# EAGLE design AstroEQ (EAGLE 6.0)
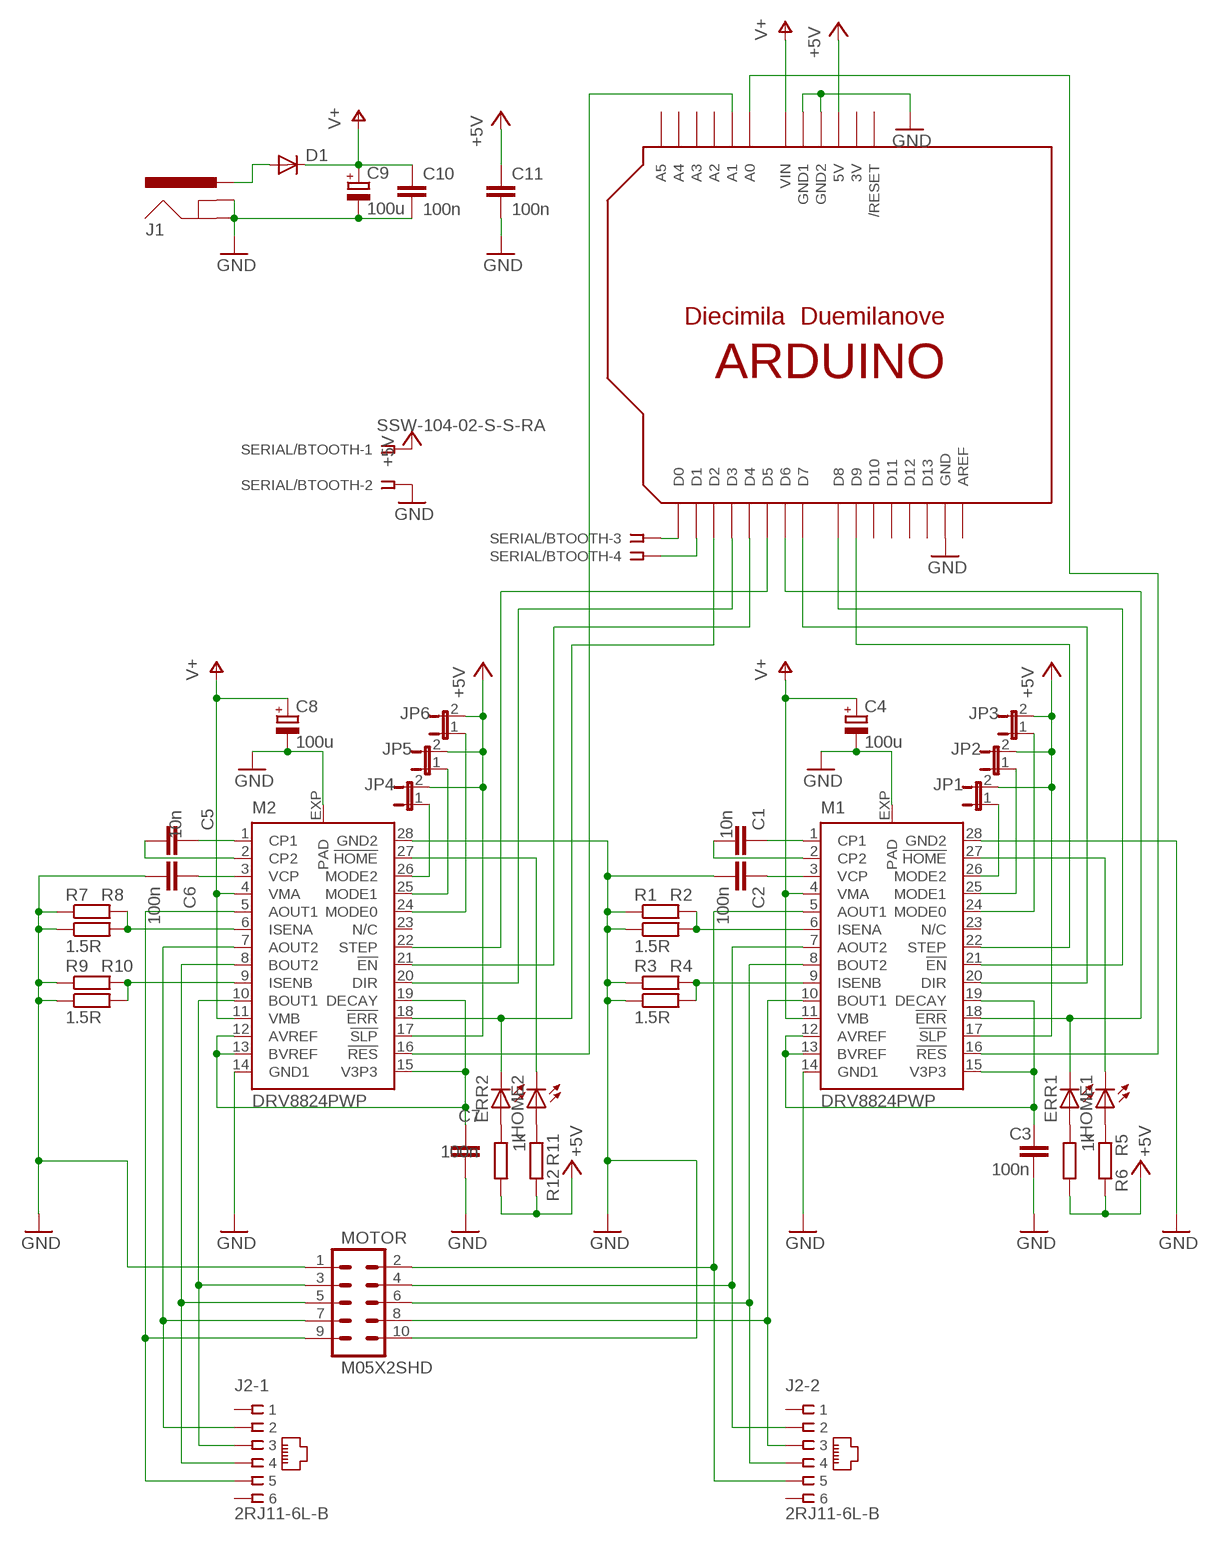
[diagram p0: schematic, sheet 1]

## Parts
C1  10n  C-EUC0603K  [C0603K]
C2  100n  C-EUC0603K  [C0603K]
C3  100n  C-EUC0603K  [C0603K]
C4  100u  CPOL-EUC/6032-28R  [C/6032-28R]
C5  10n  C-EUC0603K  [C0603K]
C6  100n  C-EUC0603K  [C0603K]
C7  100n  C-EUC0603K  [C0603K]
C8  100u  CPOL-EUC/6032-28R  [C/6032-28R]
C9  100u  CPOL-EUC/6032-28R  [C/6032-28R]
C10  100n  C-EUC0603K  [C0603K]
C11  100n  C-EUC0603K  [C0603K]
D1  DIODESMA-ALT  [SMA-DIODE_ALT]
ERR1  LEDCHIP-LED0603  [CHIP-LED0603]
ERR2  LEDCHIP-LED0603  [CHIP-LED0603]
HOME1  LEDCHIP-LED0603  [CHIP-LED0603]
HOME2  LEDCHIP-LED0603  [CHIP-LED0603]
J1  POWER_JACKPTH  [POWER_JACK_PTH]
J2  2RJ11-6L-B  [2RJ11]
JP1  JUMPER-2SMD-NO  [SJ_2S-NO]
JP2  JUMPER-2SMD-NO  [SJ_2S-NO]
JP3  JUMPER-2SMD-NO  [SJ_2S-NO]
JP4  JUMPER-2SMD-NO  [SJ_2S-NO]
JP5  JUMPER-2SMD-NO  [SJ_2S-NO]
JP6  JUMPER-2SMD-NO  [SJ_2S-NO]
M1  DRV8824PWP  [HTSSOP28PWP]
M2  DRV8824PWP  [HTSSOP28PWP]
MOTOR  M05X2SHD  [2X5-SHROUDED]
R1  1.5R  R-EU_R2512  [R2512]
R2  1.5R  R-EU_R2512  [R2512]
R3  1.5R  R-EU_R2512  [R2512]
R4  1.5R  R-EU_R2512  [R2512]
R5  1k  R-EU_R0603  [R0603]
R6  1k  R-EU_R0603  [R0603]
R7  1.5R  R-EU_R2512  [R2512]
R8  1.5R  R-EU_R2512  [R2512]
R9  1.5R  R-EU_R2512  [R2512]
R10  1.5R  R-EU_R2512  [R2512]
R11  1k  R-EU_R0603  [R0603]
R12  1k  R-EU_R0603  [R0603]
SERIAL/BTOOTH  SSW-104-02-S-S-RA  [SSW-104-02-S-S-RA]
U$1  ARDUINOUNO  [ARDUINO]

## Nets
3.3V-1: C3.1 M1.12(AVREF) M1.13(BVREF) M1.15(V3P3) M1.19(DECAY)
3.3V-2: C7.1 M2.12(AVREF) M2.13(BVREF) M2.15(V3P3) M2.19(DECAY)
!EN-1: M1.21(!EN) U$1.D8
!EN-2: M2.21(!EN) U$1.D4
!ERR-1: M1.16(!RES) U$1.A0
!ERR-2: ERR2.C M2.18(!ERR) U$1.D2
!HOME-1: HOME1.C M1.27(!HOME)
!HOME-2: HOME2.C M2.27(!HOME)
!RST-1: ERR1.C M1.18(!ERR) U$1.D6
!RST-2: M2.16(!RES) U$1.A1
+5V: C11.1 JP1.2 JP2.2 JP3.2 JP4.2 JP5.2 JP6.2 M1.17(!SLP) M2.17(!SLP) R5.2 R6.2 R11.2 R12.2 SERIAL/BTOOTH.1 U$1.5V
A1-1: J2.2-5 M1.5(AOUT1) MOTOR.2
A1-2: J2.1-5 M2.5(AOUT1) MOTOR.9
A2-1: J2.2-2 M1.7(AOUT2) MOTOR.4
A2-2: J2.1-2 M2.7(AOUT2) MOTOR.7
B1-1: J2.2-3 M1.10(BOUT1) MOTOR.8
B1-2: J2.1-3 M2.10(BOUT1) MOTOR.3
B2-1: J2.2-4 M1.8(BOUT2) MOTOR.6
B2-2: J2.1-4 M2.8(BOUT2) MOTOR.5
CP1-1: C1.1 M1.1(CP1)
CP1-2: C5.1 M2.1(CP1)
CP2-1: C1.2 M1.2(CP2)
CP2-2: C5.2 M2.2(CP2)
DIR-1: M1.20(DIR) U$1.D7
DIR-2: M2.20(DIR) U$1.D3
GND: C2.2 C3.2 C4.- C6.2 C7.2 C8.- C9.- C10.2 C11.2 J1.GND J1.GNDBREAK M1.14(GND1) M1.28(GND2) M1.EXP(PAD) M2.14(GND1) M2.28(GND2) M2.EXP(PAD) MOTOR.1 MOTOR.10 R1.1 R2.1 R3.1 R4.1 R7.1 R8.1 R9.1 R10.1 SERIAL/BTOOTH.2 U$1.GND U$1.GND1 U$1.GND2
ISENA-1: M1.6(ISENA) R1.2 R2.2
ISENA-2: M2.6(ISENA) R7.2 R8.2
ISENB-1: M1.9(ISENB) R3.2 R4.2
ISENB-2: M2.9(ISENB) R9.2 R10.2
LED1: ERR1.A R6.1
LED2: HOME1.A R5.1
LED3: ERR2.A R12.1
LED4: HOME2.A R11.1
M0-1: JP3.1 M1.24(MODE0)
M0-2: JP6.1 M2.24(MODE0)
M1-1: JP2.1 M1.25(MODE1)
M1-2: JP5.1 M2.25(MODE1)
M2-1: JP1.1 M1.26(MODE2)
M2-2: JP4.1 M2.26(MODE2)
N$7: D1.A J1.PWR
RX: SERIAL/BTOOTH.3 U$1.D0
STEP-1: M1.22(STEP) U$1.D9
STEP-2: M2.22(STEP) U$1.D5
TX: SERIAL/BTOOTH.4 U$1.D1
V+: C4.+ C8.+ C9.+ C10.1 D1.C M1.4(VMA) M1.11(VMB) M2.4(VMA) M2.11(VMB) U$1.VIN
VCP-1: C2.1 M1.3(VCP)
VCP-2: C6.1 M2.3(VCP)
Unconnected: J2.1-1 J2.1-6 J2.2-1 J2.2-6 M1.23(N/C) M2.23(N/C) U$1.A2 U$1.A3 U$1.A4 U$1.A5 U$1.AREF U$1.D10 U$1.D11 U$1.D12 U$1.D13 U$1.RESET(/RESET)

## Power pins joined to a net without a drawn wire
3V: U$1.3V

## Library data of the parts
C1-C3 C5-C7 C10 C11 = resistor:C-EU: CAPACITOR, European symbol
C4 C8 C9 = resistor:CPOL-EU: POLARIZED CAPACITOR, European symbol
D1 = SparkFun:DIODE: Diode
ERR1 ERR2 HOME1 HOME2 = led:LED: LED
J1 = SparkFun:POWER_JACK: Power Jack This is the standard 5.5mm barrel jack for power. The PTH is the most common, proven, reliable, footprint. All others are experimental. The Slot footprint only works if the mill layer is transmitted to the PCB fab house so be warned. Spark Fun Electronics SKU : PRT-00119. Mating wall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
J2 = con-tycoelectronics:2RJ11-6L-B: CORCOM Modular RJ Jacks L - Ganged Series Source: www.tycoelectronics.com .. ENG_DS_1654001_1099_RJ_L_0507.pdf; MF: TYCO ELECTRONICS; MPN: 2RJ11-6L-B; OC_FARNELL: unknown; OC_NEWARK: 48F3954
JP1-JP6 = SparkFun:JUMPER-2: Jumper
M1 M2 = texas:DRV8824
MOTOR = SparkFun:M05X2: Header 5x2 Standard 10-pin dual row 0.1" header. Commonly used with AVR-ISP. Use with Spark Fun Electronics SKU: PRT-00778
R1-R12 = resistor:R-EU_: RESISTOR, European symbol
SERIAL/BTOOTH = con-samtec:SSW-104-02-S-S: THROUGH-HOLE .025" SQ POST SOCKET Source: Samtec SSW.pdf; MPN: SSW-104-02-S-S-RA; OC_FARNELL: unknown; OC_NEWARK: 11P9385
U$1 = adafruit:ARDUINO: Arduino Diecimila/Duemilanove Make a shield with ease, this package has all the named pins as well as the two mounting drill holes and an outline of the USB and DC power connector. The outline is on the DIMENSION layer, so if your board house uses it they will cut the outline to match.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

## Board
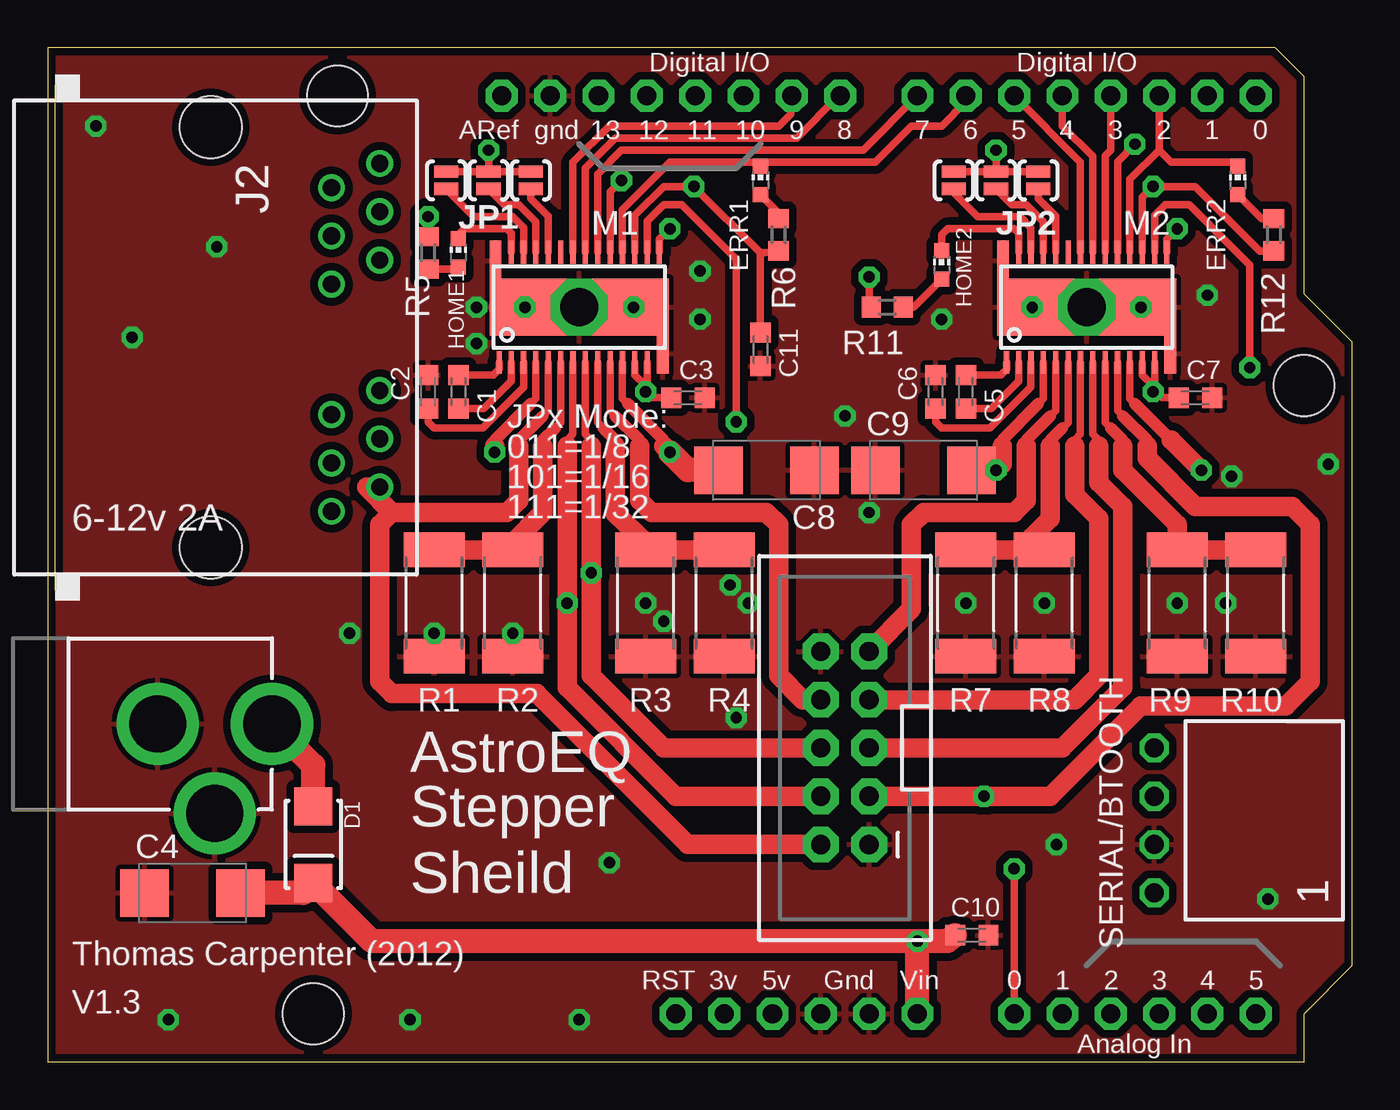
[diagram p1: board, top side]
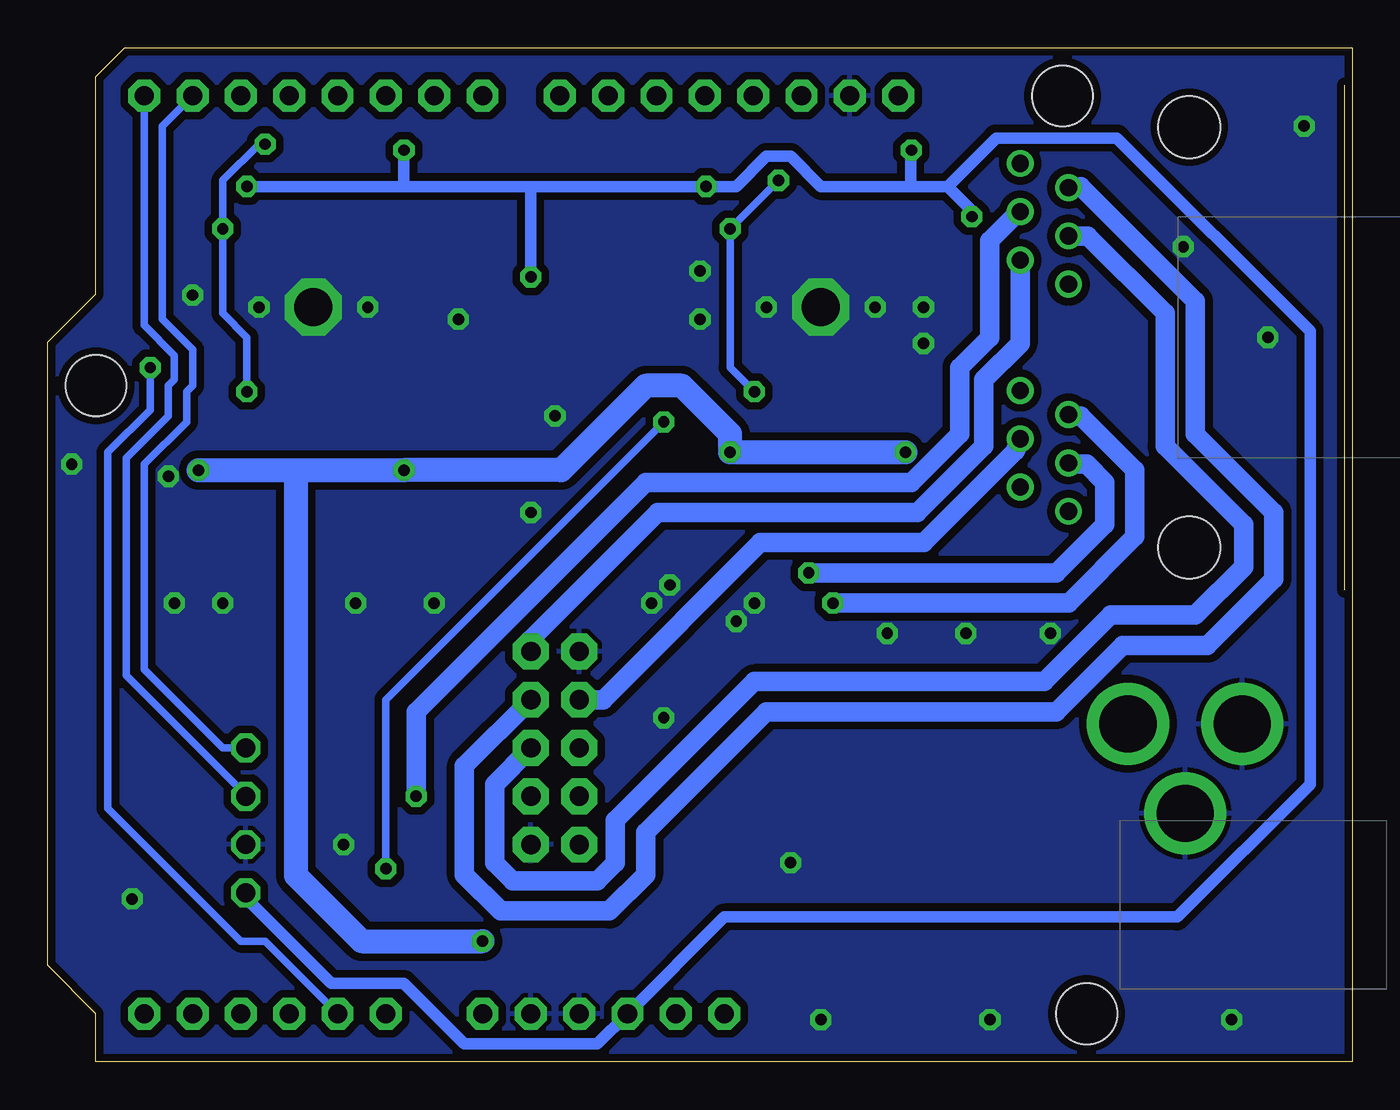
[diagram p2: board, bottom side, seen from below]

Size 68.58 x 53.34 mm. Coordinates in mm from the lower left corner, seen from the top.
Copper layers (1*16): Top 0.035mm / dielectric 1.5mm / Bottom 0.035mm
Design rules: minimum track width 0.2mm, minimum drill 0.4mm, track to track 0.2mm, track to pad 0.2mm, pad to pad 0.2mm, via to via 0.2mm, smd to smd 0mil, copper to edge 10mil, drill to drill 0.2mm, minimum pad ring 10mil, minimum via ring 10mil, stop-mask expansion 0.125mm, vias tented up to drill 0mil, thermal gap 10mil

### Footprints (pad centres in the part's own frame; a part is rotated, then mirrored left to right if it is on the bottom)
C0603K = smd 1.05 x 1.08: 1 -0.875,0; 2 0.875,0
C/6032-28R = smd 2.55 x 2.5: + 2.525,0; - -2.525,0
SMA-DIODE_ALT = smd 2 x 2: A -2,0; C 2,0
CHIP-LED0603 = smd 0.8 x 0.8: A 0,-0.75; C 0,0.75
POWER_JACK_PTH = drill 2.997 pad 4.318: GND 0,7.7; GNDBREAK 4.7,10.7; PWR 0,13.7
2RJ11 = drill 0.9 pad 1.4: 1-1 -9.144,8.89; 1-2 -7.874,6.35; 1-3 -6.604,8.89; 1-4 -5.334,6.35; 1-5 -4.064,8.89; 1-6 -2.794,6.35; 2-1 2.794,8.89; 2-2 4.064,6.35; 2-3 5.334,8.89; 2-4 6.604,6.35; 2-5 7.874,8.89; 2-6 9.144,6.35 | hole 3.251: -11.049,0; 11.049,0
SJ_2S-NO = smd 0.635 x 1.27: 1 -0.45,0; 2 0.45,0
HTSSOP28PWP = smd 0.27 x 1.2: 1 -4.21,-2.9; 2 -3.575,-2.9; 3 -2.925,-2.9; 4 -2.275,-2.9; 5 -1.625,-2.9; 6 -0.975,-2.9; 7 -0.325,-2.9; 8 0.325,-2.9; 9 0.975,-2.9; 10 1.625,-2.9; 11 2.275,-2.9; 12 2.925,-2.9; 13 3.575,-2.9; 15 4.21,2.9; 16 3.575,2.9; 17 2.925,2.9; 18 2.275,2.9; 19 1.625,2.9; 20 0.975,2.9; 21 0.325,2.9; 22 -0.325,2.9; 23 -0.975,2.9; 24 -1.625,2.9; 25 -2.275,2.9; 26 -2.925,2.9; 27 -3.575,2.9 | smd 0.61 x 2.1: 14 4.395,-2.45; 28 -4.395,2.45 | smd 9.4 x 3: EXP 0,0
2X5-SHROUDED = drill 1.016 pad 1.88 octagon: 1 -1.27,5.08; 2 1.27,5.08; 3 -1.27,2.54; 4 1.27,2.54; 5 -1.27,0; 6 1.27,0; 7 -1.27,-2.54; 8 1.27,-2.54; 9 -1.27,-5.08; 10 1.27,-5.08
R2512 = smd 1.8 x 3.2: 1 -2.8,0; 2 2.8,0
R0603 = smd 1 x 1.1: 1 -0.85,0; 2 0.85,0
SSW-104-02-S-S-RA = drill 1 pad 1.5 octagon: 1 -3.81,1.524; 2 -1.27,1.524; 3 1.27,1.524; 4 3.81,1.524
ARDUINO = drill 1 pad 1.676 octagon: 3V 35.56,2.54; 5V 38.1,2.54; A0 50.8,2.54; A1 53.34,2.54; A2 55.88,2.54; A3 58.42,2.54; A4 60.96,2.54; A5 63.5,2.54; AREF 23.876,50.8; D0 63.5,50.8; D1 60.96,50.8; D2 58.42,50.8; D3 55.88,50.8; D4 53.34,50.8; D5 50.8,50.8; D6 48.26,50.8; D7 45.72,50.8; D8 41.656,50.8; D9 39.116,50.8; D10 36.576,50.8; D11 34.036,50.8; D12 31.496,50.8; D13 28.956,50.8; GND 26.416,50.8; GND1 43.18,2.54; GND2 40.64,2.54; RESET 33.02,2.54; VIN 45.72,2.54 | hole 3.2: 15.24,50.8; 66.04,35.56; 13.97,2.54

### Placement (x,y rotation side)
C1  21.59,35.24 270 top
C2  20,35.24 90 top
C3  33.66,34.92 0 top
C4  7.62,8.89 0 top
C5  48.26,35.24 270 top
C6  46.67,35.24 90 top
C7  60.33,34.92 0 top
C8  37.78,31.11 180 top
C9  46.04,31.11 0 top
C10  48.58,6.67 0 top
C11  37.47,37.47 270 top
D1  13.97,11.43 270 top
ERR1  37.47,46.35 0 top
ERR2  62.55,46.35 0 top
HOME1  21.59,42.55 0 top
HOME2  46.99,41.91 0 top
J1  -1.91,17.78 270 top
J2  8.57,38.1 270 top
JP1  20.95,46.35 90 top
JP2  23.18,46.35 90 top
JP3  25.4,46.35 90 top
JP4  47.62,46.35 90 top
JP5  49.85,46.35 90 top
JP6  52.07,46.35 90 top
M1  27.94,39.69 0 top
M2  54.61,39.69 0 top
MOTOR  41.91,16.51 180 top
R1  20.32,24.13 90 top
R2  24.45,24.13 90 top
R3  31.43,24.13 90 top
R4  35.56,24.13 90 top
R5  20,42.55 90 top
R6  38.42,43.5 270 top
R7  48.26,24.13 90 top
R8  52.39,24.13 90 top
R9  59.37,24.13 90 top
R10  63.5,24.13 90 top
R11  44.13,39.69 180 top
R12  64.45,43.5 270 top
SERIAL/BTOOTH  59.69,12.7 90 top
U$1  0,0 0 top

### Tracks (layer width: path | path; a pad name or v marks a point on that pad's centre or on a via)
3.3V-1  (via drill 0.6)
  Top 0.406: M1.19 29.57,45.76 v30.16,46.35 | M1.12 30.86,36.13 31.43,35.56 v31.43,35.24 | M1.13 31.52,35.33 v31.43,35.24 | M1.15 32.15,43.26 v32.7,43.81 | v31.43,35.24 31.75,34.92 C3.1
  Bottom 0.406: v31.43,35.24 32.7,36.51 v32.7,43.81 v30.16,46.35
3.3V-2  (via drill 0.6)
  Top 0.406: M2.19 56.23,47.34 v57.15,48.26 | M2.12 57.53,36.13 58.1,35.56 v58.1,35.24 58.19,35.33 | M2.13 58.19,35.33 | M2.15 58.82,43.26 v59.37,43.81 | 58.19,35.33 58.59,34.92 C7.1
  Bottom 0.406: v57.15,48.26 57.47,48.26 59.37,46.35 v59.37,43.81 59.37,39.37 58.1,38.1 v58.1,35.24
!EN-1
  Top 0.406: M1.21 28.27,47 29.84,48.58 39.37,48.58 41.59,50.8 U$1.D8
!EN-2
  Top 0.406: M2.21 54.94,47.62 53.34,49.21 U$1.D4
!ERR-1  (via drill 0.6)
  Top 0.406: M1.16 31.52,44.22 32.38,45.09 33.34,45.09 36.2,42.23 v36.2,33.66 | v50.8,10.16 U$1.A0
  Bottom 0.406: v36.2,33.66 50.8,19.05 v50.8,10.16
!ERR-2
  Top 0.406: M2.18 56.88,46.41 58.42,47.94 | 58.42,47.94 U$1.D2 | 58.42,47.94 59.05,47.31 62.23,47.31 ERR2.C
!HOME-1
  Top 0.406: M1.27 24.36,43.58 24.13,43.81 21.91,43.81 21.59,43.5 HOME1.C
!HOME-2
  Top 0.406: M2.27 51.03,43.58 50.8,43.81 47.31,43.81 46.99,43.5 HOME2.C
!RST-1
  Top 0.406: M1.18 30.21,44.82 32.7,47.31 37.15,47.31 | 37.15,47.31 43.5,47.31 45.4,49.21 46.99,49.21 48.26,50.48 U$1.D6 | ERR1.C 37.15,47.31
!RST-2  (via drill 0.6)
  Top 0.406: M2.16 58.19,44.53 58.74,45.09 60.01,45.09 63.18,41.91 v63.18,36.51
  Bottom 0.406: v63.18,36.51 63.18,34.29 65.41,32.07 65.41,13.34 58.42,6.35 57.15,6.35 U$1.A1
+5V  (via drill 0.6)
  Top 0.406: M1.17 30.86,44.52 32.38,46.04 v33.97,46.04 37.47,42.55 | M2.17 57.53,45.47 v58.1,46.04 60.33,46.04 63.72,42.65 R12.2 | JP4.2 JP5.2 | JP6.2 JP5.2 | JP5.2 v49.85,47.94 | JP1.2 JP2.2 | JP3.2 JP2.2 | JP2.2 v23.18,47.94 | 37.47,42.55 C11.1 | R6.2 37.68,42.55 37.47,42.55 | R5.2 v20,44.45 | R11.2 43.18,39.79 v43.18,41.27
  Bottom 0.61: 43.18,46.04 v33.97,46.04 32.38,46.04 30.8,47.62 29.53,47.62 27.94,46.04 23.21,46.04 | 43.18,46.04 49.85,46.04 | 49.85,46.04 v58.1,46.04 | v49.85,47.94 49.85,46.04 | 23.21,46.04 21.27,46.04 | 23.21,46.04 23.21,47.91 v23.18,47.94 | v43.18,41.27 43.18,46.04 | 21.27,46.04 18.73,48.58 12.38,48.58 2.22,38.42 2.22,14.61 9.21,7.62 33.02,7.62 U$1.5V 39.69,0.95 46.67,0.95 49.85,4.13 53.66,4.13 58.17,8.64 SERIAL/BTOOTH.1 | 21.27,46.04 20,44.77 v20,44.45
A1-1
  Top 0.406: M1.5 26.32,34.25 26.04,33.97 | 24.77,32.38 24.77,32.7
  Top 0.61: 26.04,33.97 24.77,32.7
  Top 1.016: 18.1,28.89 17.46,28.26 17.46,20 18.1,19.37 25.72,19.37 33.66,11.43 MOTOR.2 | 18.1,28.89 24.13,28.89 24.77,29.53 24.77,32.38 | J2.2-5 16.76,30.23 18.1,28.89
A1-2
  Top 0.406: M2.5 52.98,34.25 52.7,33.97 | 51.44,32.7 51.44,32.38
  Top 0.61: 52.7,33.97 51.44,32.7
  Top 1.016: 51.44,32.38 51.44,29.53 50.8,28.89 46.04,28.89 45.4,28.26 45.4,23.81 MOTOR.9
  Bottom 1.016: J2.1-5 17.46,37.78 19.37,35.88 19.37,32.38 22.86,28.89 36.51,28.89 43.18,22.23 MOTOR.9
A2-1  (via drill 0.6)
  Top 0.406: M1.7 27.61,33.01 27.3,32.7 27.3,32.38
  Top 1.016: 27.3,32.38 v27.3,24.13 27.3,19.68 33.02,13.97 MOTOR.4
  Bottom 1.016: v27.3,24.13 14.92,24.13 11.43,27.62 11.43,31.11 14.29,33.97 14.92,33.97 J2.2-2
A2-2
  Top 0.406: M2.7 54.28,33.01 53.98,32.7 53.98,32.38
  Top 1.016: 53.98,32.38 53.98,29.84 55.24,28.57 55.24,20.32 53.98,19.05 MOTOR.7
  Bottom 1.016: J2.1-2 14.29,46.04 8.26,40.01 8.26,33.02 4.13,28.89 4.13,25.4 7.62,21.91 12.06,21.91 15.56,18.41 30.8,18.41 37.15,12.06 37.15,9.84 39.05,7.94 44.77,7.94 46.67,9.84 46.67,15.56 MOTOR.7
B1-1
  Top 0.406: M1.10 29.57,34.25 29.84,33.97 | 31.11,32.7 31.11,32.38
  Top 0.61: 29.84,33.97 31.11,32.7
  Top 1.016: 31.11,32.38 31.11,29.53 31.75,28.89 37.78,28.89 38.42,28.26 38.42,20.32 39.69,19.05 MOTOR.8
  Bottom 1.016: J2.2-3 17.72,32.13 22.54,27.3 31.11,27.3 39.37,19.05 MOTOR.8
B1-2  (via drill 0.6)
  Top 0.406: M2.10 56.23,34.25 56.52,33.97 | 57.78,32.7 57.78,32.38
  Top 0.61: 56.52,33.97 57.78,32.7
  Top 1.016: 57.78,32.38 57.78,31.75 60.33,29.21 65.41,29.21 66.36,28.26 66.36,20 65.09,18.73 57.47,18.73 52.7,13.97 v49.21,13.97 MOTOR.3
  Bottom 1.016: J2.1-3 17.53,44.7 19.05,43.18 19.05,38.1 20.64,36.51 20.64,33.02 23.18,30.48 37.15,30.48 49.21,18.41 v49.21,13.97
B2-1  (via drill 0.6)
  Top 0.406: M1.8 28.27,33.01 28.57,32.7 28.57,32.38
  Top 1.016: 28.57,32.38 v28.57,25.72 28.57,20.32 32.38,16.51 MOTOR.6
  Bottom 1.016: v28.57,25.72 15.56,25.72 13.02,28.26 13.02,30.48 13.97,31.43 14.54,31.43 J2.2-4
B2-2
  Top 0.406: M2.8 54.94,33.01 55.24,32.7 55.24,32.38
  Top 1.016: 55.24,32.38 55.24,30.48 56.52,29.21 56.52,19.68 53.34,16.51 MOTOR.5
  Bottom 1.016: J2.1-4 13.91,43.43 9.84,39.37 9.84,32.38 5.71,28.26 5.71,26.04 8.26,23.5 12.7,23.5 16.19,20 31.43,20 38.73,12.7 38.73,10.48 39.69,9.53 44.13,9.53 45.09,10.48 45.09,14.61 MOTOR.5
CP1-1
  Top 0.406: M1.1 23.73,36.43 23.42,36.12 C1.1
CP1-2
  Top 0.406: M2.1 50.4,36.43 50.09,36.12 C5.1
CP2-1
  Top 0.406: M1.2 24.36,35.8 22.94,34.37 C1.2
CP2-2
  Top 0.406: M2.2 51.03,35.8 49.61,34.37 C5.2
DIR-1
  Top 0.406: U$1.D7 42.86,47.94 30.16,47.94 28.91,46.7 M1.20
DIR-2
  Top 0.406: M2.20 55.59,47.65 55.88,47.94 U$1.D3
GND  (via drill 0.6, 2)
  other vias: 20.32,22.54 24.45,22.54 31.43,24.13 36.83,24.13 25.08,39.69 30.8,39.69 51.75,39.69 57.47,39.69 48.26,24.13 52.39,24.13 59.37,24.13 61.91,24.13 54.61,39.69 27.94,39.69 64.14,8.57 53.02,11.43 29.53,10.48 4.45,38.1 8.89,42.86 2.54,49.21 19.05,2.22 27.94,2.22 6.35,2.22 67.31,31.43 62.23,30.8 43.18,28.89 41.91,33.97 46.99,39.05 60.96,40.32 34.29,39.05 34.29,41.59 22.54,37.78 22.54,39.69 35.88,25.08 32.38,23.18 36.2,18.1 15.88,22.54
  pour Bottom (isolate 0.406): 0,53.34 68.58,53.34 68.58,0 0,0
  pour Top (isolate 0.406): 0,53.34 68.58,53.34 68.58,0 0,0
ISENA-1
  Top 0.406: M1.6 26.96,33.63 26.67,33.34 | 26.04,32.7 26.04,32.38
  Top 0.61: 26.67,33.34 26.04,32.7
  Top 1.016: R1.2 R2.2 24.39,27.25 26.04,28.89 26.04,32.38
ISENA-2
  Top 0.406: M2.6 53.63,33.63 53.34,33.34 | 52.7,32.7 52.7,32.38
  Top 0.61: 53.34,33.34 52.7,32.7
  Top 1.016: R7.2 R8.2 51.7,27.57 52.7,28.57 52.7,32.38
ISENB-1
  Top 0.406: M1.9 28.91,33.63 29.21,33.34 | 29.84,32.7 29.84,32.38
  Top 0.61: 29.21,33.34 29.84,32.7
  Top 1.016: R4.2 R3.2 31.43,27.3 29.84,28.84 29.84,32.38
ISENB-2
  Top 0.406: M2.9 55.59,33.63 55.88,33.34 | 56.52,32.7 56.52,32.38
  Top 0.61: 55.88,33.34 56.52,32.7
  Top 1.016: R10.2 R9.2 59.37,28.26 56.52,31.11 56.52,32.38
LED1
  Top 0.406: ERR1.A 38.62,44.45 38.42,44.45 R6.1
LED2
  Top 0.406: HOME1.A 21.39,41.59 21.59,41.91 21.59,41.7 R5.1
LED3
  Top 0.406: ERR2.A 63.8,44.35 R12.1
LED4
  Top 0.406: HOME2.A 45.52,39.69 R11.1
M0-1
  Top 0.406: M1.24 26.32,44.49 25.4,45.4 JP3.1
M0-2
  Top 0.406: M2.24 52.98,44.49 52.07,45.4 JP6.1
M1-1
  Top 0.406: M1.25 25.66,44.19 24.77,45.09 24,45.09 JP2.1
M1-2
  Top 0.406: M2.25 52.34,44.19 51.44,45.09 50.67,45.09 JP5.1
M2-1
  Top 0.406: M1.26 25.02,43.88 24.45,44.45 22.41,44.45 JP1.1
M2-2
  Top 0.406: M2.26 51.69,43.88 51.12,44.45 48.9,44.45 47.94,45.4 47.62,45.72 JP4.1
N$7
  Top 1.27: D1.A 13.97,15.61 J1.PWR
RX
  Bottom 0.406: SERIAL/BTOOTH.3 58.17,14.03 64.45,20.32 64.45,31.75 62.23,33.97 62.23,35.56 61.91,35.88 61.91,37.15 63.5,38.73 U$1.D0
STEP-1
  Top 0.406: M1.22 27.61,47.3 29.53,49.21 38.42,49.21 39.05,49.85 39.05,50.74 U$1.D9
STEP-2
  Top 0.406: M2.22 54.28,47.31 U$1.D5
TX
  Bottom 0.406: SERIAL/BTOOTH.4 59.37,16.51 63.5,20.64 63.5,31.43 61.28,33.66 61.28,35.24 60.96,35.56 60.96,37.47 62.55,39.05 62.55,49.21 U$1.D1
V+  (via drill 0.6)
  Top 0.305: M1.4 25.66,35.83 | M1.11 30.21,35.83
  Top 0.406: M1.4 25.66,34.87 25.4,34.61 | M2.4 52.34,34.87 52.07,34.61 | M2.11 56.88,34.87 57.15,34.61 | M1.11 30.21,34.87 30.48,34.61 | 23.5,32.7 23.5,32.38 | 50.16,32.7 50.16,32.38 | 32.38,32.38 32.38,32.7
  Top 0.61: 25.4,34.61 23.5,32.7 | 52.07,34.61 50.16,32.7 | 30.48,34.61 32.38,32.7 | 57.15,34.61 59.05,32.7
  Top 1.016: C9.+ v49.85,31.11 50.16,31.43 50.16,32.38 | v23.5,32.07 23.5,32.38 | v32.7,32.07 32.38,32.38 | v60.64,31.11 59.05,32.7
  Top 1.27: C4.+ 13.43,8.89 D1.C 17.05,6.35 v45.72,6.35 | U$1.VIN v45.72,6.35 | C10.1 47.38,6.43 47.31,6.35 v45.72,6.35 | C8.+ 33.66,31.11 v32.7,32.07
  Bottom 1.27: v60.64,31.11 55.53,31.11 | 55.53,31.11 v49.85,31.11 41.59,31.11 37.15,35.56 35.24,35.56 32.7,33.02 v32.7,32.07 v23.5,32.07 | 55.53,31.11 55.53,9.81 52.07,6.35 v45.72,6.35
VCP-1
  Top 0.406: M1.3 25.02,35.49 22.86,33.34 20.32,33.34 20,33.66 C2.1
VCP-2
  Top 0.406: M2.3 51.69,35.49 49.53,33.34 46.99,33.34 46.67,33.66 C6.1

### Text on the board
tNames: JP1 | JP2 | JPx Mode: | 011=1/8 | 101=1/16 | 111=1/32 | 6-12v 2A | AstroEQ | Stepper | Sheild | Thomas Carpenter (2012) | V1.3
tDocu: Free | Free

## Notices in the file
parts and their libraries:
SparkFun: Licensing: CC v3.0 Share-Alike You are welcome to use this library for commercial purposes.
